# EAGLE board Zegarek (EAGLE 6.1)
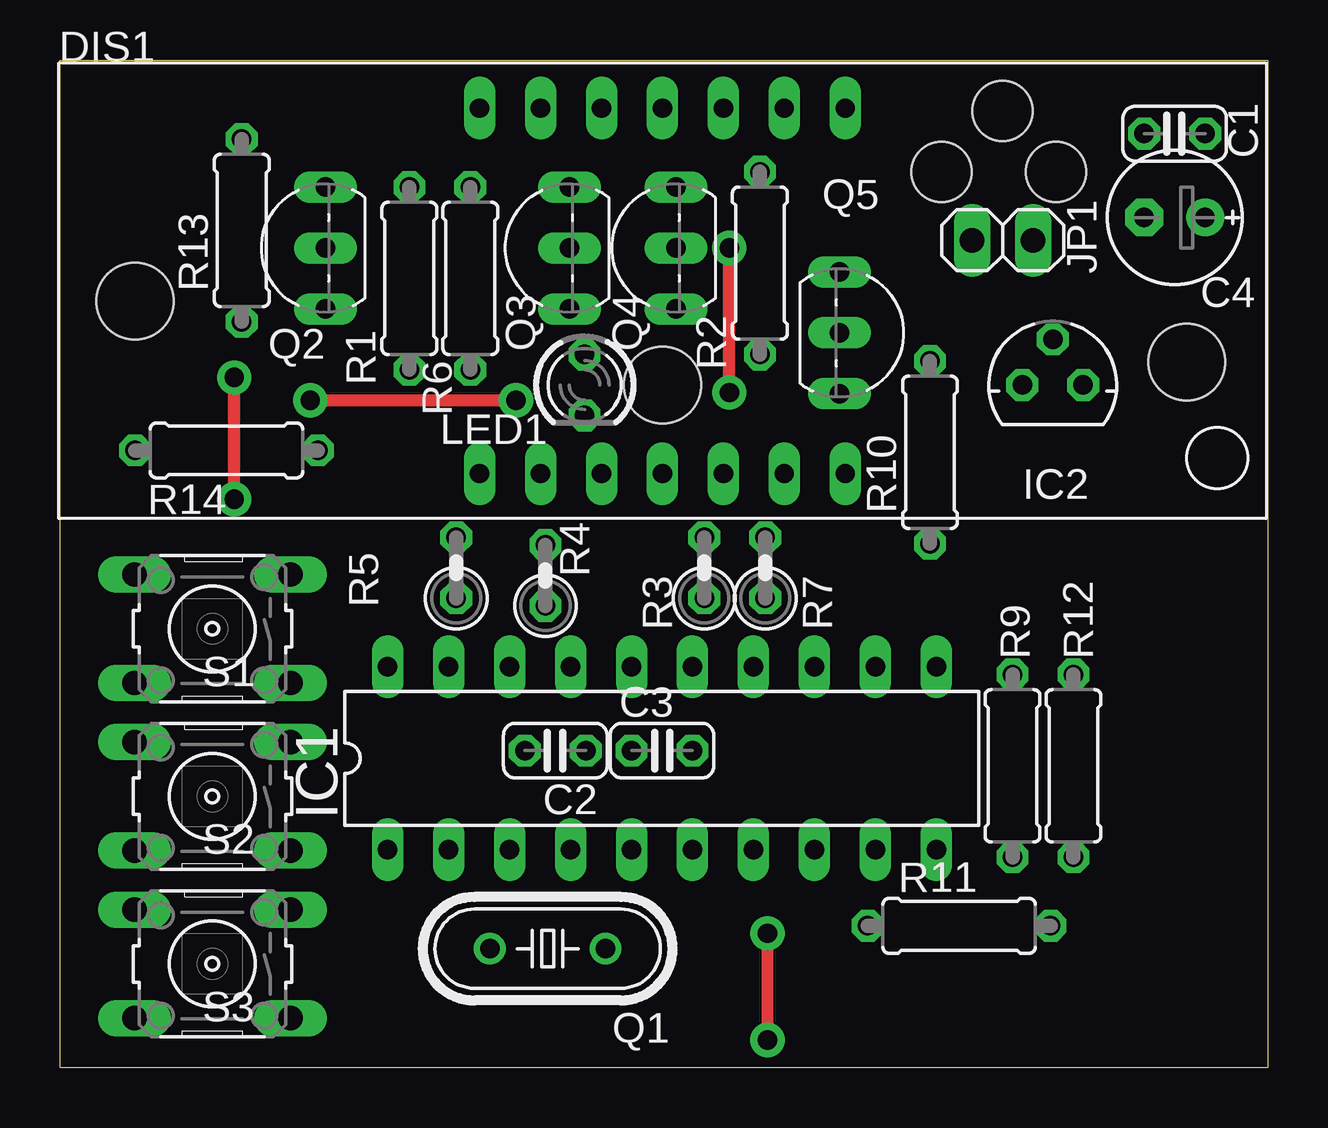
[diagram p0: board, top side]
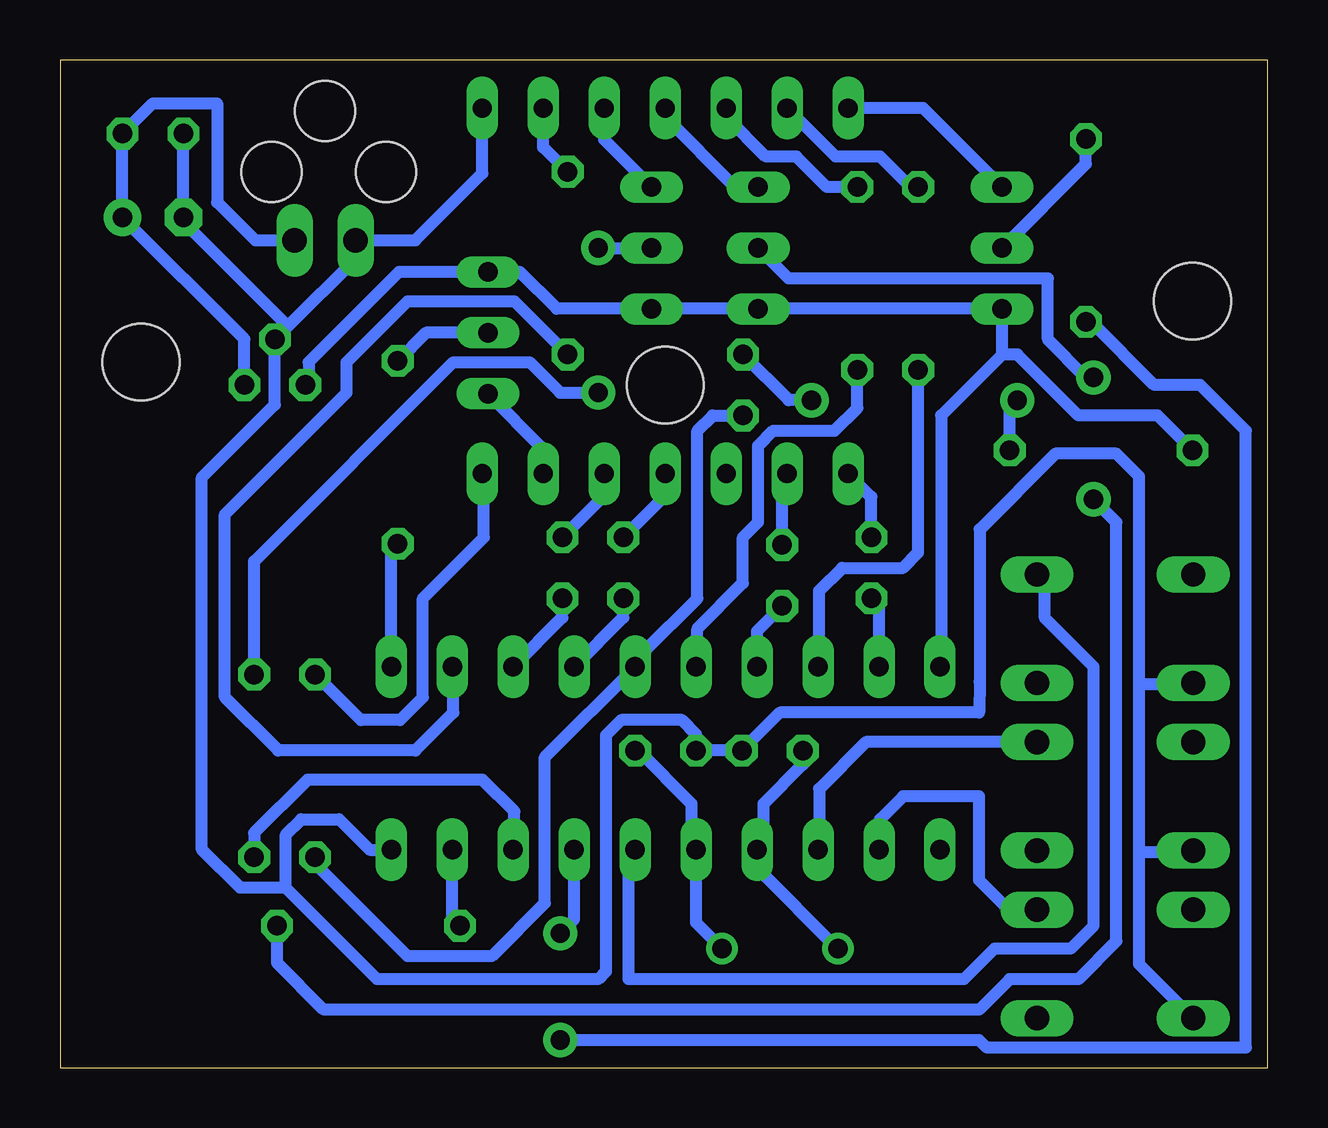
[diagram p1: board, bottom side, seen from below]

Size 50.32 x 42 mm. Coordinates in mm from the lower left corner, seen from the top.
Outline: 0,42 50.32,42 50.32,0 0,0 0,42
Copper layers (1*16): Top 0.035mm / dielectric 1.5mm / Bottom 0.035mm
Design rules: minimum track width 20mil, minimum drill 24mil, track to track 8mil, track to pad 8mil, pad to pad 8mil, via to via 8mil, smd to smd 8mil, copper to edge 5mil, drill to drill 8mil, minimum pad ring 10mil, minimum via ring 8mil, stop-mask expansion 4mil, vias tented up to drill 0mil, thermal gap 10mil
Holes 2.5 mm at 36.73,37.34 41.5,37.34 39.27,39.88
Holes 3.2 mm at 25.1,28.45 46.94,29.4 3.13,31.94

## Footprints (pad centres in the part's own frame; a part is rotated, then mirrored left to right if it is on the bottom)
C025-024X044 = drill 0.813 octagon: 1 -1.27,0; 2 1.27,0
E2,5-6E = drill 0.813 pad 1.575: + -1.27,0 | drill 0.813 pad 1.575 octagon: - 1.27,0
4X14.2CA = drill 0.8 pad 1.27 long: 1 17.53,1.88; 2 20.07,1.88; 3 22.61,1.88; 4 25.15,1.88; 5 27.69,1.88; 6 30.23,1.88; 7 32.77,1.88; 8 32.77,17.12; 9 30.23,17.12; 10 27.69,17.12; 11 25.15,17.12; 12 22.61,17.12; 13 20.07,17.12; 14 17.53,17.12
DIL20 = drill 0.813 long: 1 -11.43,-3.81; 2 -8.89,-3.81; 3 -6.35,-3.81; 4 -3.81,-3.81; 5 -1.27,-3.81; 6 1.27,-3.81; 7 3.81,-3.81; 8 6.35,-3.81; 9 8.89,-3.81; 10 11.43,-3.81; 11 11.43,3.81; 12 8.89,3.81; 13 6.35,3.81; 14 3.81,3.81; 15 1.27,3.81; 16 -1.27,3.81; 17 -3.81,3.81; 18 -6.35,3.81; 19 -8.89,3.81; 20 -11.43,3.81
78LXX = drill 0.813 octagon: GND 0,1.905; IN 1.27,0; OUT -1.27,0
1X02 = drill 1.016 long: 1 -1.27,0; 2 1.27,0
LED3MM = drill 0.813 octagon: A -1.27,0; K 1.27,0
HC49/S = drill 0.813: 1 -2.413,0; 2 2.413,0
TO92-EBC = drill 0.813 long: B 0,-1.27; C -2.54,-1.27; E 2.54,-1.27
0207/7 = drill 0.813 octagon: 1 -3.81,0; 2 3.81,0
0207/2V = drill 0.813 octagon: 1 -1.27,0; 2 1.27,0
B3F-10XX = drill 1.016 long: 1 -3.251,2.261; 2 3.251,2.261; 3 -3.251,-2.261; 4 3.251,-2.261

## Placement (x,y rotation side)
C1  100n  [C025-024X044]  46.45,38.93 180 top
C2  27p  [C025-024X044]  20.64,13.21 180 top
C3  27p  [C025-024X044]  25.08,13.21 0 top
C4  100u  [E2,5-6E]  46.45,35.44 180 top
DIS1  [4X14.2CA]  -0.05,22.88 0 top
IC1  ATTiny2313  [DIL20]  25.08,12.89 0 top
IC2  78L05  [78LXX]  41.37,28.45 0 top
JP1  Supply  [1X02]  39.27,34.48 0 top
LED1  [LED3MM]  21.86,28.45 270 top
Q1  8MHz  [HC49/S]  20.32,4.96 180 top
Q2  BC546B  [TO92-EBC]  9.79,34.16 90 top
Q3  BC546B  [TO92-EBC]  19.96,34.16 90 top
Q4  BC546B  [TO92-EBC]  24.4,34.16 90 top
Q5  BC546B  [TO92-EBC]  33.75,30.62 270 top
R1  470  [0207/7]  14.56,32.9 90 top
R2  470  [0207/7]  29.16,33.53 90 top
R3  470  [0207/2V]  26.84,20.83 90 top
R4  470  [0207/2V]  20.23,20.51 90 top
R5  470  [0207/2V]  16.51,20.83 90 top
R6  470  [0207/7]  17.1,32.9 90 top
R7  470  [0207/2V]  29.39,20.83 90 top
R9  220  [0207/7]  39.69,12.58 270 top
R10  4k7  [0207/7]  36.25,25.64 90 top
R11  4k7  [0207/7]  37.47,5.91 0 top
R12  4k7  [0207/7]  42.23,12.58 90 top
R13  4k7  [0207/7]  7.57,34.9 90 top
R14  470  [0207/7]  6.93,25.72 180 top
S1  SET  [B3F-10XX]  6.35,18.29 180 top
S2  +  [B3F-10XX]  6.35,11.31 180 top
S3  -  [B3F-10XX]  6.35,4.32 180 top

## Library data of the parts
C1-C4 R1-R7 R9-R14 = rcl
DIS1 = led-7-segment
IC1 = atmel
IC2 = v-reg
JP1 = pinhead
LED1 = led
Q1 = crystal
Q2-Q5 = transistor-npn
S1-S3 = switch-omron

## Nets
A: IC1.18 R1.1
A1: Q2.B R13.2
A2: Q3.B R11.2
A3: Q4.B R12.2
A4: Q5.B R10.2
B: IC1.12 R2.1
C: IC1.14 R3.1
D: IC1.17 R4.1
DT: IC1.15 LED1.K R9.2
E: IC1.19 R5.1
F: IC1.16 R6.1
G: IC1.13 R7.1
GND: C1.2 C2.1 C3.1 C4.- DIS1.8 IC1.10 IC2.GND JP1.1 S1.2 S2.2 S3.2
N$1: DIS1.13 R1.2
N$2: DIS1.9 R2.2
N$3: DIS1.4 R3.2
N$4: DIS1.2 R4.2
N$5: DIS1.1 R5.2
N$6: DIS1.12 R6.2
N$7: DIS1.5 R7.2
N$8: IC1.11 R10.1
N$9: DIS1.7 R9.1
N$10: DIS1.6 Q5.E
N$11: DIS1.10 Q4.E
N$12: DIS1.11 Q3.E
N$13: DIS1.14 Q2.E
N$14: IC1.9 R11.1
N$15: IC1.8 R12.1
N$16: IC1.7 R13.1
N$17: IC1.6 S1.3
N$18: IC1.3 S2.3
N$19: IC1.2 S3.3
N$20: C1.1 C4.+ IC2.IN JP1.2
N$21: C2.2 IC1.4 Q1.2
N$22: C3.2 IC1.5 Q1.1
N$24: LED1.A R14.1
VCC: IC1.20 IC2.OUT Q2.C Q3.C Q4.C Q5.C R14.2

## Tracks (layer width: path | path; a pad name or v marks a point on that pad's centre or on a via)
A
  Bottom 0.508: R1.1 14.56,21.47 15.19,20.83 17.73,20.83 18.69,19.88 18.69,16.75 IC1.18
A1
  Bottom 0.508: R13.2 7.57,37.66 Q2.B
A2  (via drill 0.8 pad 1.42)
  Top 0.508: v7.26,23.69 v7.26,28.77
  Bottom 0.508: R11.2 41.27,4.37 39.32,2.42 12.02,2.42 10.75,3.69 7.89,3.69 6.3,5.27 6.3,22.74 v7.26,23.69 | Q3.B 19.96,32.9 9.16,32.9 9.16,30.36 7.57,28.77 v7.26,28.77
A3  (via drill 0.8 pad 1.42)
  Top 0.508: v27.89,28.13 v27.89,34.16
  Bottom 0.508: v27.89,28.13 29.48,28.13 30.75,29.4 33.92,29.4 42.23,21.1 R12.2 | v27.89,34.16 Q4.B
A4
  Bottom 0.508: R10.2 35.08,30.63 Q5.B
B
  Bottom 0.508: R2.1 31.39,31.94 35.83,31.94 38.37,29.4 38.37,28.13 43.45,23.05 43.45,15.43 41.23,13.21 35.51,13.21 33.92,14.8 33.92,16.65 IC1.12
C
  Bottom 0.508: R3.1 26.84,18.75 IC1.14
D
  Bottom 0.508: IC1.17 21.27,18.2 R4.1
DT
  Bottom 0.508: R9.2 39.69,8.5 35.83,4.64 32.34,4.64 30.12,6.86 30.12,12.94 IC1.15 25.99,17.07 25.99,17.34 23.76,19.56 23.76,26.54 23.13,27.18 LED1.K
E
  Bottom 0.508: IC1.19 16.19,19.24 R5.1
F
  Bottom 0.508: R6.1 17.1,27.5 18.05,26.54 20.59,26.54 21.23,25.91 21.23,22.74 21.86,22.1 21.86,20.2 23.76,18.29 23.76,16.75 IC1.16
G
  Bottom 0.508: R7.1 29.39,18.75 IC1.13
GND
  Bottom 0.508: IC1.10 37.42,9.08 38.69,10.35 40.27,10.35 40.91,9.72 40.91,7.5 | S3.2 5.35,4.31 5.35,9 | 5.35,9 5.35,16 | S1.2 3.13,16 5.35,16 | S2.2 3.14,9 5.35,9 | 40.91,7.5 37.1,3.69 27.89,3.69 27.57,4 27.57,13.84 26.94,14.48 24.4,14.48 23.81,13.89 C3.1 C2.1 20.32,14.8 12.02,14.8 12,16.09 12,22.43 8.84,25.59 6.3,25.59 5.35,24.64 5.35,16 | 40.82,30.9 IC2.GND 41.37,27.63 44.4,24.6 44.4,9.08 42.81,7.5 40.91,7.5 | 40.82,30.9 38.01,33.72 JP1.1 35.51,34.48 32.72,37.27 DIS1.8 | C1.2 C4.- 45.17,35.25 40.82,30.9
N$1
  Bottom 0.508: R1.2 14.87,36.71 16.14,37.97 18,37.97 DIS1.13
N$2
  Bottom 0.508: DIS1.9 30.18,38.36 R2.2
N$3
  Bottom 0.508: DIS1.4 25.1,23.84 R3.2
N$4
  Bottom 0.508: R4.2 20.23,24.55 DIS1.2
N$5
  Bottom 0.508: R5.2 16.51,23.78 DIS1.1
N$6
  Bottom 0.508: DIS1.12 22.56,39.63 20.91,37.97 19.64,37.97 18.37,36.71 R6.2
N$7
  Bottom 0.508: DIS1.5 27.64,23.84 R7.2
N$8
  Bottom 0.508: IC1.11 36.51,21.57 R10.1
N$9
  Bottom 0.508: R9.1 37.78,14.48 36.15,14.48 35.19,15.43 35.19,19.56 32.66,22.1 32.66,24.69 DIS1.7
N$10
  Bottom 0.508: DIS1.6 30.18,25.79 Q5.E
N$11
  Bottom 0.508: DIS1.10 27.64,38.68 Q4.E
N$12
  Bottom 0.508: DIS1.11 25.1,39.63 22.18,36.71 Q3.E
N$13
  Bottom 0.508: Q2.E 14.35,40 DIS1.14
N$14
  Bottom 0.508: IC1.9 33.97,6.22 R11.1
N$15
  Bottom 0.508: IC1.8 31.39,9.13 31.39,10.67 32.72,12 40,12 42.23,9.77 R12.1
N$16  (via drill 0.8 pad 1.42)
  Top 0.508: v29.48,1.15 v29.48,5.59
  Bottom 0.508: IC1.7 28.89,6.18 v29.48,5.59 | v29.48,1.15 12.02,1.15 11.7,0.83 0.91,0.83 0.91,26.54 2.81,28.45 4.72,28.45 7.35,31.08 R13.1
N$17
  Bottom 0.508: IC1.6 26.62,8.81 26.62,3.69 12.65,3.69 11.38,4.96 8.21,4.96 7.26,5.91 7.26,16.7 9.28,18.73 9.28,20.23 S1.3
N$18
  Bottom 0.508: S2.3 16.74,13.57 18.69,11.62 18.69,9.13 IC1.3
N$19
  Bottom 0.508: S3.3 10.79,6.58 12.02,7.81 12.02,11.31 15.19,11.31 16.14,10.35 16.14,9.13 IC1.2
N$20
  Bottom 0.508: JP1.2 42.18,34.48 43.77,36.07 43.77,40.2 46.44,40.2 C1.1 C4.+ 42.63,30.36 IC2.IN
N$21
  Bottom 0.508: C2.2 19.37,12.63 21,11 21,9.35 IC1.4 21.27,8.32 Q1.2
N$22
  Bottom 0.508: C3.2 26.21,13.21 24,11 24,9.27 IC1.5 23.81,6.03 Q1.1
N$24  (via drill 0.8 pad 1.42)
  Top 0.508: v10.43,27.81 v19,27.81
  Bottom 0.508: R14.1 10.75,27.5 v10.43,27.81 | v19,27.81 19.96,27.81 LED1.A
VCC
  Bottom 0.508: 11.07,29.72 Q2.C Q3.C Q4.C 29.62,31.63 31.16,33.16 Q5.C 36.19,33.16 39.96,29.4 39.96,28.59 IC2.OUT | 11.07,29.72 13.6,27.18 13.6,16.75 IC1.20 | R14.2 4.58,27.18 7.89,27.18 10.43,29.72 11.07,29.72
